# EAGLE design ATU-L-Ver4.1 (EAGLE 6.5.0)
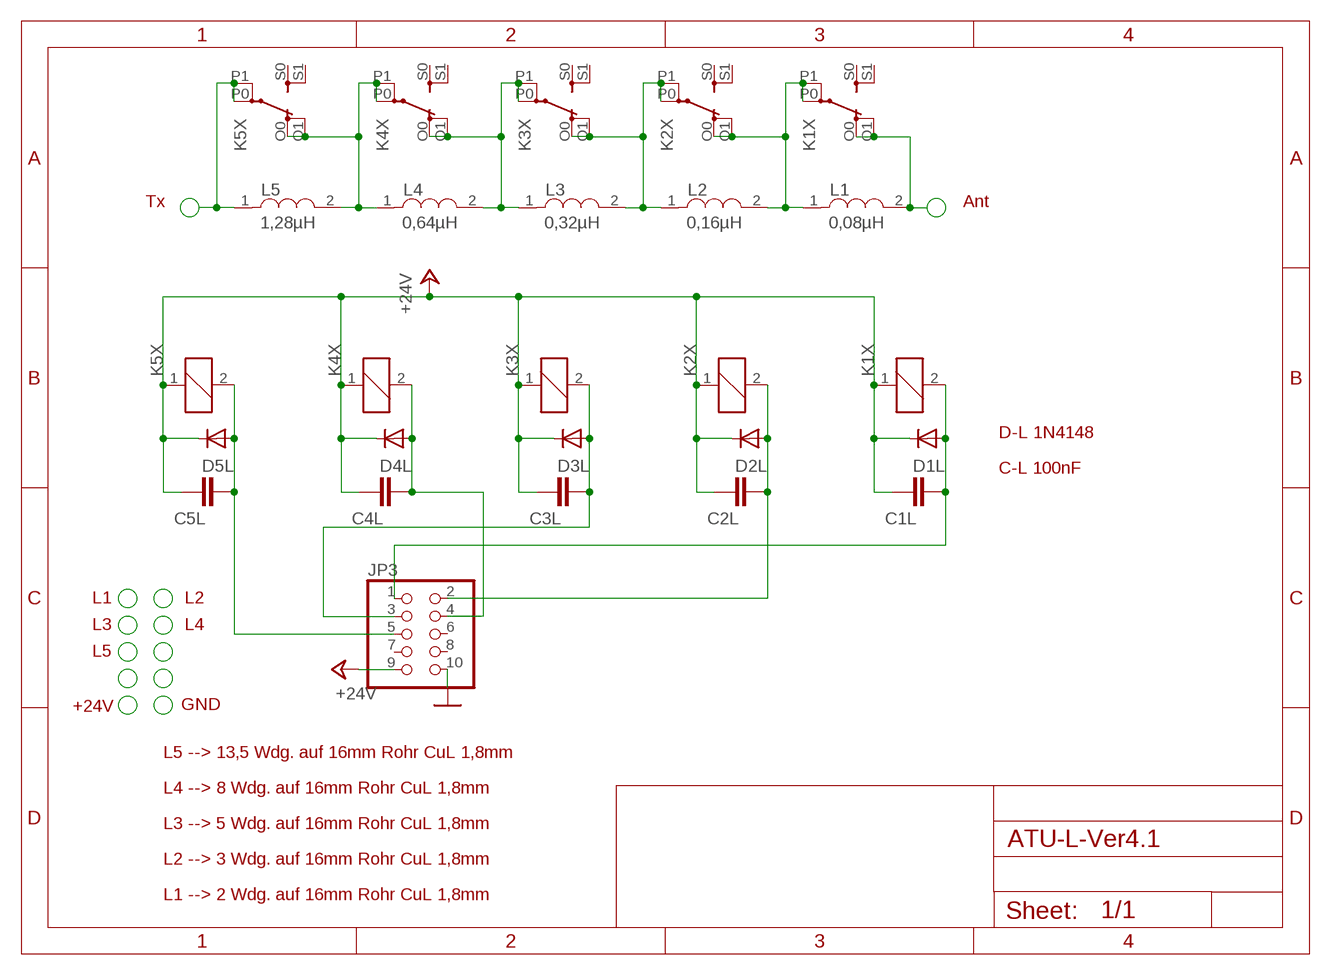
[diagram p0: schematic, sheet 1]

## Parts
C1L  C-EUC1206  [C1206]
C2L  C-EUC1206  [C1206]
C3L  C-EUC1206  [C1206]
C4L  C-EUC1206  [C1206]
C5L  C-EUC1206  [C1206]
D1L  DIODE-MINIMELF  [MINIMELF]
D2L  DIODE-MINIMELF  [MINIMELF]
D3L  DIODE-MINIMELF  [MINIMELF]
D4L  DIODE-MINIMELF  [MINIMELF]
D5L  DIODE-MINIMELF  [MINIMELF]
JP3  PINHD-2X5  [2X05]
K1X  G2RE  [G2R2E]
K2X  G2RE  [G2R2E]
K3X  G2RE  [G2R2E]
K4X  G2RE  [G2R2E]
K5X  G2RE  [G2R2E]
L1  0,08µH  LUFTSPULE0,2µH  [LUFTSPULE0,2µH]
L2  0,16µH  LUFTSPULE0,2µH  [LUFTSPULE0,2µH]
L3  0,32µH  LUFTSPULE0,4µH  [LUFTSPULE0,4µH]
L4  0,64µH  LUFTSPULE0,8µH  [LUFTSPULE0,8µH]
L5  1,28µH  1,2µH_STEHEND  [1,2µH_STEHEND]

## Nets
+24V: C1L.1 C2L.1 C3L.1 C4L.1 C5L.1 D1L.C D2L.C D3L.C D4L.C D5L.C JP3.9 K1X.1 K2X.1 K3X.1 K4X.1 K5X.1
GND: JP3.10
LX-1: C1L.2 D1L.A JP3.1 K1X.2
LX-2: C2L.2 D2L.A JP3.2 K2X.2
LX-3: C3L.2 D3L.A JP3.3 K3X.2
LX-4: C4L.2 D4L.A JP3.4 K4X.2
LX-5: C5L.2 D5L.A JP3.5 K5X.2
N$1: K1X.P0(P) K1X.P1(P) K2X.O0(O) K2X.O1(O) L1.1 L2.2
N$2: K1X.O0(O) K1X.O1(O) L1.2
N$14: K4X.P0(P) K4X.P1(P) K5X.O0(O) K5X.O1(O) L4.1 L5.2
N$34: K2X.P0(P) K2X.P1(P) K3X.O0(O) K3X.O1(O) L2.1 L3.2
N$35: K3X.P0(P) K3X.P1(P) K4X.O0(O) K4X.O1(O) L3.1 L4.2
N$58: K5X.P0(P) K5X.P1(P) L5.1
Unconnected: JP3.6 JP3.7 JP3.8 K1X.S0(S) K1X.S1(S) K2X.S0(S) K2X.S1(S) K3X.S0(S) K3X.S1(S) K4X.S0(S) K4X.S1(S) K5X.S0(S) K5X.S1(S)

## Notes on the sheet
- Tx | Ant
- D-L 1N4148
- C-L 100nF
- L1 | L2
- L3 | L4
- L5
- +24V | GND
- L5 --> 13,5 Wdg. auf 16mm Rohr CuL 1,8mm
- L4 --> 8 Wdg. auf 16mm Rohr CuL 1,8mm
- L3 --> 5 Wdg. auf 16mm Rohr CuL 1,8mm
- L2 --> 3 Wdg. auf 16mm Rohr CuL 1,8mm
- L1 --> 2 Wdg. auf 16mm Rohr CuL 1,8mm

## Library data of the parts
C1L C2L C3L C4L C5L = rcl:C-EU: CAPACITOR, European symbol
D1L D2L D3L D4L D5L = diode:DIODE-: DIODE
JP3 = pinhead:PINHD-2X5: PIN HEADER
K1X K2X K3X K4X K5X = EIGEN_2:G2RE
L1 L2 = EIGEN_2:LUFTSPULE0,2µH: Luftspule N=3 auf 16mm Installationsrohr,
L3 = EIGEN_2:LUFTSPULE0,4µH: Luftspule N=5 auf 16mm Installationsrohr,
L4 = EIGEN_2:LUFTSPULE0,8µH: uftspule N=7 auf 16mm Installationsrohr,
L5 = dk3ha-2020:1,2µH_STEHEND: 1,2µH - 1,6µ stehende Montage

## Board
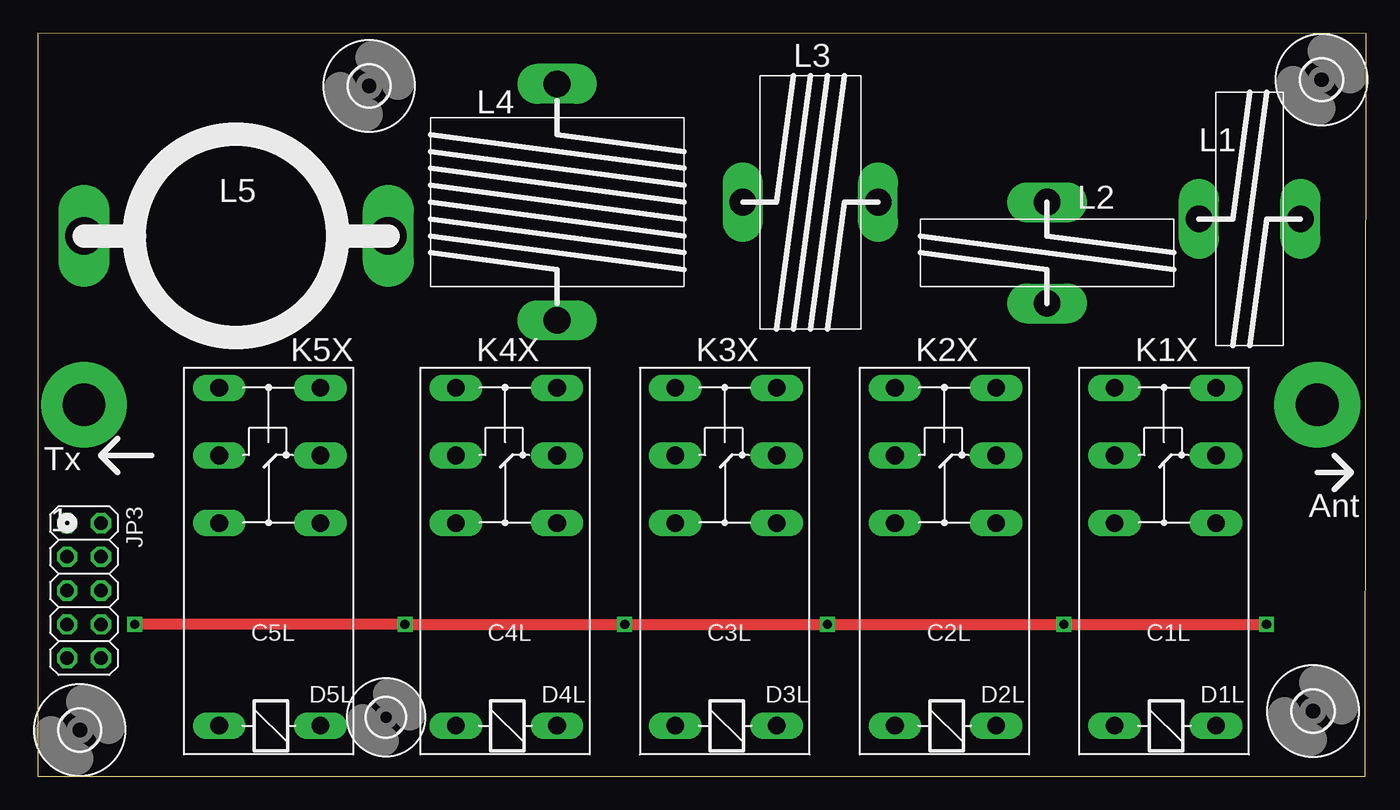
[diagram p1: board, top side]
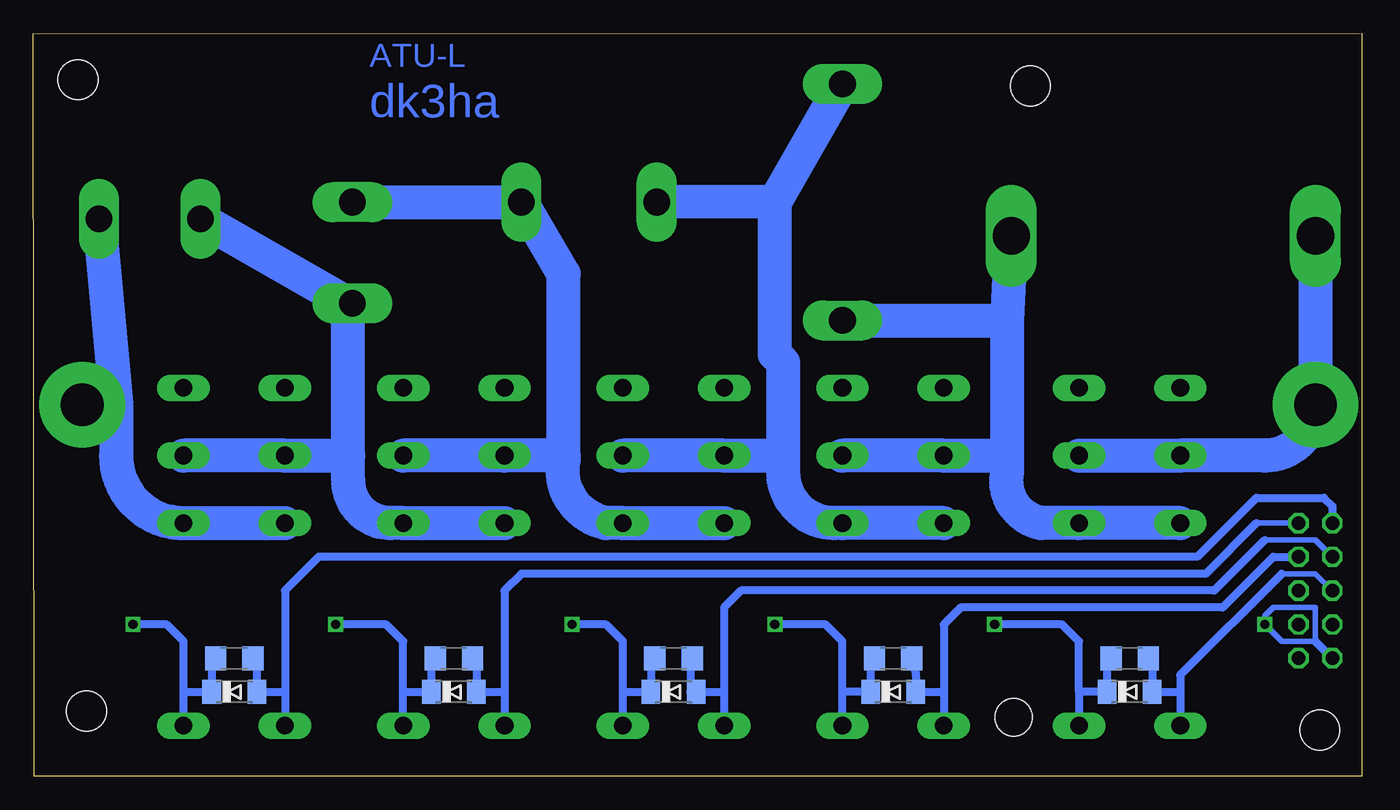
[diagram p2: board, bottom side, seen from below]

Size 99.88 x 55.88 mm. Coordinates in mm from the lower left corner, seen from the top.
Outline: 0,55.88 0,0 99.83,0.03 99.88,55.84 0,55.88
Copper layers (1*16): Top 0.035mm / dielectric 1.5mm / Bottom 0.035mm
Design rules "default": minimum track width 10mil, minimum drill 24mil, track to track 8mil, track to pad 8mil, pad to pad 8mil, via to via 8mil, smd to smd 8mil, copper to edge 40mil, drill to drill 8mil, minimum pad ring 10mil, minimum via ring 8mil, stop-mask expansion 4mil, vias tented up to drill 0mil, thermal gap 10mil

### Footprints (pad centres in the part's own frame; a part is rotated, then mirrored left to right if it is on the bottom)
C1206 = smd 1.6 x 1.8: 1 -1.4,0; 2 1.4,0
MINIMELF = smd 1.4 x 1.8: A 1.7,0; C -1.7,0
2X05 = drill 1.016 octagon: 1 -5.08,-1.27; 2 -5.08,1.27; 3 -2.54,-1.27; 4 -2.54,1.27; 5 0,-1.27; 6 0,1.27; 7 2.54,-1.27; 8 2.54,1.27; 9 5.08,-1.27; 10 5.08,1.27
G2R2E = drill 1.321 long: 1 -12.7,-3.81; 2 -12.7,3.81; O0 2.54,-3.81; O1 2.54,3.81; P0 7.62,-3.81; P1 7.62,3.81; S0 12.7,-3.81; S1 12.7,3.81
LUFTSPULE0,2µH = drill 2 long: 1 -3.81,0; 2 3.81,0
LUFTSPULE0,4µH = drill 2 long: 1 -5.08,0; 2 5.08,0
LUFTSPULE0,8µH = drill 2 long: 1 -8.89,0; 2 8.89,0
1,2µH_STEHEND = drill 2.8 long: 1 -11.43,0; 2 11.43,0
3,0 = hole 3: 0,0
2,8 = hole 2.8: 0,0

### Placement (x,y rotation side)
C1L  84.77,8.89 0 bottom
C2L  68.26,8.89 0 bottom
C3L  51.75,8.89 0 bottom
C4L  35.24,8.89 0 bottom
C5L  17.46,8.89 0 bottom
D1L  84.77,6.35 0 bottom
D2L  68.26,6.35 0 bottom
D3L  51.75,6.35 0 bottom
D4L  35.24,6.35 0 bottom
D5L  17.46,6.35 0 bottom
JP3  3.49,13.97 270 top
K1X  84.77,16.51 90 top
K2X  68.26,16.51 90 top
K3X  51.75,16.51 90 top
K4X  35.24,16.51 90 top
K5X  17.46,16.51 90 top
L1  91.12,41.91 0 top
L2  75.88,39.37 270 top
L3  58.1,43.18 0 top
L4  39.05,43.18 90 top
L5  14.92,40.64 0 top
U$1  [3,0]  3.18,3.49 0 top
U$2  [3,0]  95.89,4.92 0 top
U$3  [3,0]  96.52,52.39 0 top
U$4  [3,0]  24.92,51.91 0 top
U$5  [2,8]  26.19,4.45 0 top

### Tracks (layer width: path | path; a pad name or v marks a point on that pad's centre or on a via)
+24V  (via drill 0.7)
  Top 0.813: v92.39,11.43 v77.15,11.43 v59.37,11.43 v44.13,11.43 v27.62,11.43 v7.3,11.43
  Bottom 0.406: 3.49,10.16 6.03,10.16 v7.3,11.43 7.3,12.06 6.67,12.7 3.49,12.7 3.49,10.16
  Bottom 0.61: 21.27,6.35 K5X.1 | JP3.9 3.49,10.16 | 21.27,6.35 21.27,10.16 22.54,11.43 v27.62,11.43 | 21.27,6.35 D5L.C 19.16,8.89 C5L.1 | C4L.1 36.94,8.89 D4L.C | C3L.1 53.45,8.89 D3L.C 55.56,6.35 | C2L.1 69.96,8.89 D2L.C 72.07,6.35 | C1L.1 86.47,8.89 D1L.C 88.58,6.35 | K4X.1 39.05,6.35 | 39.05,6.35 39.05,10.16 40.32,11.43 v44.13,11.43 | D4L.C 39.05,6.35 | D4L.C 36.51,6.35 | K3X.1 55.56,6.35 | 55.56,6.35 55.56,10.16 56.83,11.43 v59.37,11.43 | K2X.1 72.07,6.35 | 72.07,6.35 72.07,10.16 73.34,11.43 v77.15,11.43 | K1X.1 88.58,6.35 | 88.58,6.35 88.58,10.16 89.85,11.43 v92.39,11.43
LX-1
  Bottom 0.61: 80.96,6.35 80.96,13.97 78.42,16.51 12.38,16.51 7.94,20.95 2.86,20.95 2.22,20.32 JP3.1 | 80.96,6.35 K1X.2 | C1L.2 83.07,8.89 D1L.A 80.96,6.35
LX-2
  Bottom 0.406: 7.94,19.05 JP3.2
  Bottom 0.61: 64.45,6.35 64.45,13.97 63.18,15.24 11.75,15.24 7.94,19.05 | 64.45,6.35 K2X.2 | 64.45,6.35 D2L.A 66.56,8.89 C2L.2
LX-3
  Bottom 0.406: 7.3,17.78 3.49,17.78 JP3.3
  Bottom 0.61: 47.94,6.35 47.94,12.7 46.67,13.97 11.11,13.97 7.3,17.78 | 47.94,6.35 K3X.2 | C3L.2 50.48,8.89 50.48,6.35 D3L.A 47.94,6.35
LX-4
  Bottom 0.61: 31.43,6.35 31.43,11.43 30.16,12.7 10.48,12.7 6.67,16.51 JP3.4 | 31.43,6.35 K4X.2 | 31.43,6.35 D4L.A 33.54,7.62 C4L.2
LX-5
  Bottom 0.406: JP3.5 3.49,15.24 6.03,15.24
  Bottom 0.61: 6.03,15.24 13.65,7.62 13.65,6.35 | 13.65,6.35 K5X.2 | 13.65,6.35 D5L.A 15.76,8.89 C5L.2
N$1
  Bottom 2.54: K1X.P0 K1X.P1 76.2,24.13 | K2X.O1 K2X.O0 73.02,19.05 arc90 76.2,22.23 76.2,24.13 | 76.2,24.13 76.2,35.56 | 76.2,35.56 L2.2 | 76.2,35.56 L1.1
N$2  (via drill 3.2 pad 6.45)
  Bottom 2.54: K1X.O1 K1X.O0 arc90 93.66,24.13 93.66,27.94 | L1.2 93.66,27.94 | v96.2,27.94 93.66,27.94
N$14
  Bottom 2.54: K4X.P0 K4X.P1 26.67,24.13 | K5X.O1 K5X.O0 24.13,19.05 arc90 26.67,22.86 26.67,24.13 | L4.1 26.67,34.29 | 26.67,24.13 26.67,34.29 | 26.67,34.29 L5.2
N$34
  Bottom 2.54: K2X.P0 K2X.P1 60.01,24.13 | K3X.O1 K3X.O0 56.83,19.05 arc90 60.01,23.81 60.01,24.13 | 60.01,24.13 60.01,37.78 L3.2 L2.1
N$35
  Bottom 2.54: K4X.O1 K4X.O0 39.69,19.05 arc90 43.5,22.86 43.5,24.13 | K3X.P0 K3X.P1 43.5,24.13 | 43.5,24.13 43.5,31.11 44.13,31.75 44.14,43.21 | 44.14,43.21 L3.1 | L4.2 44.14,43.21
N$58  (via drill 3.2 pad 6.45)
  Bottom 2.54: K5X.P0 K5X.P1 7.3,24.13 arc-90 v3.49,27.94 L5.1

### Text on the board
Bottom: ATU-L | dk3ha
tPlace: Tx | Ant | 1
